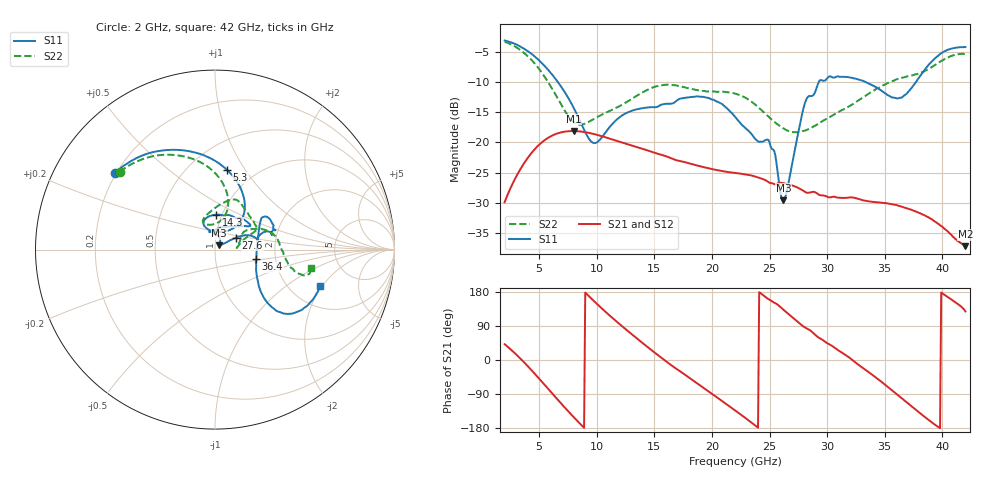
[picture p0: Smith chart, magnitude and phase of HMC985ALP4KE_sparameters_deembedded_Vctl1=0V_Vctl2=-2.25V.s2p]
!s2p File: Measurements: S11, S21, S12, S22
# GHz S dB R 50.0
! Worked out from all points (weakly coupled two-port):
!   401 points, 2 GHz to 42 GHz, reference 50 ohm
!   highest |S21| = -18.11 dB at 8 GHz (marker M1); lowest = -37.2 dB at 42 GHz (marker M2)
!   lowest |S11| = -29.6 dB at 26.2 GHz (marker M3), VSWR 1.07, Z = 52.3 + j2.45 ohm
!   |S11| at or under -10 dB: 6.635 GHz to 29.27 GHz (22.63 GHz wide, 126 % of centre); 33.37 GHz to 37.7 GHz (4.326 GHz wide, 12.2 % of centre)
!   |S22| runs from -18.3 to -3.3 dB; largest |S21 - S12| = 0.00019
!   S11 on the Smith chart (normalised r, x): 2 GHz: 0.19, +0.33; 5.3 GHz: 0.75, +0.83; 14.3 GHz: 0.94, +0.38; 27.6 GHz: 1.25, +0.17; 36.4 GHz: 1.58, -0.18; 42 GHz: 2.90, -1.91
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2  -3.06 142.6  -29.94 41.7  -29.94 41.7  -3.28 140.8
3.5  -4.22 115.6  -24.04 -0.2  -24.04 -0.2  -4.85 112.9
5.3  -6.96 81.4  -19.88 -59.6  -19.88 -59.6  -8.60 83.2
8  -14.26 47.7  -18.11 -150.9  -18.11 -150.9  -16.64 86.6
8.7  -17.09 52.3  -18.21 -172.9  -18.21 -172.9  -17.04 100.4
9.9  -20.09 88.3  -18.68 151.3  -18.68 151.3  -15.94 113.2
12.2  -15.52 112.2  -20.02 89.1  -20.02 89.1  -13.74 100.3
14.3  -14.21 88.4  -21.26 36.9  -21.27 36.9  -11.36 78.4
15.4  -13.94 73.3  -21.95 11.0  -21.95 11.0  -10.57 70.7
19.3  -12.44 34.2  -24.11 -74.1  -24.12 -74.2  -11.44 42.2
22  -15.73 52.3  -25.06 -132.8  -25.08 -132.8  -11.88 25.5
25  -20.02 98.7  -26.71 158.8  -26.72 158.8  -15.90 17.5
26.2  -29.65 45.1  -26.77 132.7  -26.77 132.7  -17.68 8.7
27.6  -17.37 29.7  -27.67 96.7  -27.65 96.6  -18.21 4.9
28.1  -13.30 20.9  -28.24 85.5  -28.23 85.5  -18.02 7.0
28.7  -12.27 13.0  -28.21 73.9  -28.21 73.9  -17.48 11.5
31  -9.06 23.3  -29.18 24.9  -29.20 25.0  -14.93 30.6
33.3  -9.94 34.2  -29.69 -25.3  -29.70 -25.4  -12.32 28.2
35.4  -12.27 12.1  -30.17 -74.3  -30.18 -74.3  -10.04 19.0
36.4  -12.58 -13.1  -30.62 -99.1  -30.63 -99.2  -9.29 13.0
39.5  -5.81 -43.4  -33.33 -174.0  -33.34 -173.8  -6.96 -14.0
42  -4.15 -19.0  -37.23 128.1  -37.22 128.0  -5.29 -10.7
